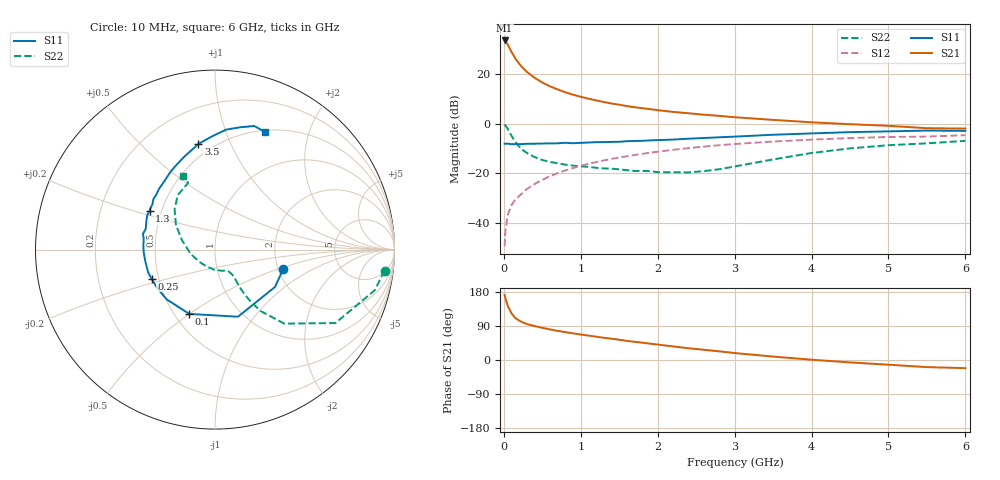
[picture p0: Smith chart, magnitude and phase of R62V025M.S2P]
! SIEMENS Small Signal Semiconductors
! BFR193
! Si NPN RF Bipolar Junction Transistor in SOT23
! VCE = 2 V  IC = 25 mA
! Common Emitter S-Parameters:  May  1996
# GHz  S  MA  R  50
!  f  S11  S21  S12  S22
! GHz  MAG  ANG  MAG  ANG  MAG  ANG  MAG  ANG
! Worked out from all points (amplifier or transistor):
!   36 points, 10 MHz to 6 GHz, reference 50 ohm
!   highest |S21| = 33.3 dB at 10 MHz (marker M1)
!   |S21| within 3 dB of that: start of sweep to 73.44 MHz
!   unconditionally stable (mu >= 1): 477.5 MHz to 1.936 GHz
!   at 250 MHz: K = 0.89, MSG = 24.9 dB, |S12| = -27.6 dB
!   at 1.4 GHz: K = 1.02, MAG = 10.1 dB, |S12| = -14.2 dB
!   at 6 GHz: K = 0.95, MSG = 1.3 dB, |S12| = -4.7 dB
!   S11 on the Smith chart (normalised r, x): 10 MHz: 2.12, -0.56; 100 MHz: 0.59, -0.50; 250 MHz: 0.46, -0.17; 1.3 GHz: 0.43, +0.23; 3.5 GHz: 0.42, +0.76; 6 GHz: 0.52, +1.38
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0.01  0.3953 -16.2  46.05 171.6  0.0035 83.7  0.9523 -7.1
0.02  0.3936 -32.0  44.87 163.4  0.0069 80.1  0.9183 -14.3
0.05  0.3952 -71.1  38.39 143.3  0.0147 69.5  0.7856 -31.4
0.1  0.3859 -111.8  27.09 122.6  0.0234 65.0  0.5648 -46.9
0.15  0.3866 -134.3  20.03 110.8  0.0299 63.7  0.4264 -53.4
0.2  0.3868 -146.6  15.7 103.8  0.0356 66.0  0.3454 -55.7
0.25  0.3886 -155.4  12.79 98.7  0.0417 66.6  0.2927 -56.5
0.3  0.3936 -161.2  10.8 95.0  0.0488 68.3  0.2573 -56.7
0.4  0.3942 -171.2  8.246 89.6  0.0616 69.6  0.2129 -56.0
0.5  0.3977 -178.1  6.616 84.9  0.0743 70.4  0.1858 -55.3
0.6  0.3999 176.9  5.567 80.7  0.0881 70.2  0.1704 -55.4
0.7  0.4017 171.4  4.811 76.9  0.1016 70.0  0.16 -56.2
0.8  0.411 167.7  4.221 73.6  0.1149 69.2  0.1499 -57.2
0.9  0.4029 163.4  3.777 70.3  0.1289 68.3  0.1436 -57.9
1.1  0.4164 156.5  3.142 64.4  0.1558 66.4  0.1354 -63.0
1.3  0.424 149.3  2.696 58.7  0.1826 63.9  0.1263 -68.0
1.7  0.4468 137.7  2.117 48.1  0.2343 58.8  0.1118 -83.9
2.2  0.4769 125.6  1.709 35.8  0.2977 51.6  0.1061 -113.3
3.5  0.5959 98.9  1.182 9.0  0.4352 31.2  0.1911 164.1
4.5  0.6717 84.6  0.97 -6.4  0.5114 17.0  0.3177 135.1
5.5  0.7226 72.4  0.806 -18.8  0.5481 2.9  0.4007 111.9
6  0.7125 66.9  0.792 -21.5  0.5833 -1.2  0.4498 113.4
